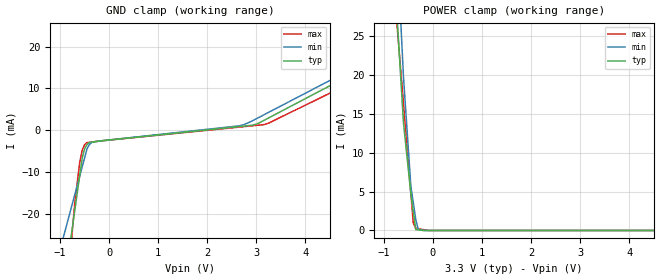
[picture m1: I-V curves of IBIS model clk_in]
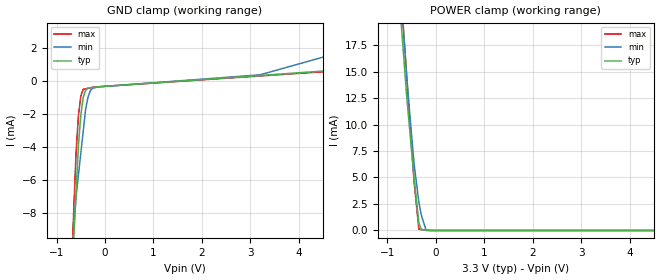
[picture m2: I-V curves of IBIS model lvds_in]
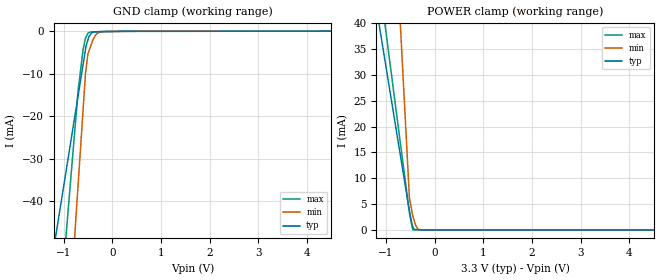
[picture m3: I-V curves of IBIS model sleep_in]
| Teraspeed (R) Labs.
| http://www.teraspeed.com
[IBIS Ver]   3.2
[Comment Char] |_char
[File Name]   dac5675aiphp.ibs
[File Rev]   3.0
[Date]   07-19-2011
[Notes]   Quality Check of this IBIS model: Model Passes IBIS Check
   Model parses into ICX IS. Simulation done with Hyperlynx.
   1. MIN TYP MAX information is based on Temprature and Voltage
   characteristics only.
   2. Package information extracted using Tektronix IConnect Software.
[Disclaimer]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
[Source]
| This model file was created by Teraspeed Consulting Group LLC
| (http://www.teraspeed.com/).
[Disclaimer]
| This product is designed as an aid for customers of Texas Instruments.
| No warranties, either expressed or implied, with respect to this third
| party software (if any) or with respect to its fitness for any
| particular purpose is claimed by Texas Instruments or the author. The
| software (if any) is provided solely on an "as is" basis. The entire
| risk as to its quality and performance is with the customer
[Copyright]
| (C) Copyright 2011 Texas Instruments Incorporated. All rights reserved.
| All other rights are reserved.
[Component]   DAC5675AIPHP
[Manufacturer] TI
[Package]
| 48-HTQFP
| variable   typ   min   max
R_pkg  1.000E-02  1.000E-02  1.000E-02
L_pkg  1.807E-09  1.620E-09  2.200E-09
C_pkg  6.730E-13  6.560E-13  7.110E-13
[Pin] signal_name  model_name  R_pin  L_pin C_pin
1   D13A   lvds_in   1.000E-02 2.200E-09 6.320E-13
2   D13B   lvds_in   1.000E-02 1.870E-09 7.110E-13
3   D12A   lvds_in   1.000E-02 1.790E-09 6.940E-13
4   D12B   lvds_in   1.000E-02 1.700E-09 6.770E-13
5   D11A   lvds_in   1.000E-02 1.660E-09 6.680E-13
6   D11B   lvds_in   1.000E-02 1.620E-09 6.560E-13
7   D10A   lvds_in   1.000E-02 1.620E-09 6.560E-13
8   D10B   lvds_in   1.000E-02 1.660E-09 6.680E-13
9   D9A   lvds_in   1.000E-02 1.700E-09 6.770E-13
10   D9B   lvds_in   1.000E-02 1.790E-09 6.940E-13
11   D8A   lvds_in   1.000E-02 1.870E-09 7.110E-13
12   D8B   lvds_in   1.000E-02 2.200E-09 6.320E-13
13   D7A   lvds_in   1.000E-02 2.200E-09 6.320E-13
14   D7B   lvds_in   1.000E-02 1.870E-09 7.110E-13
15   DVDD   POWER   1.000E-02 1.790E-09 6.940E-13
16   DGND   GND   1.000E-02 1.700E-09 6.770E-13
17   DVDD   POWER   1.000E-02 1.660E-09 6.680E-13
18   DGND   GND   1.000E-02 1.620E-09 6.560E-13
19   AGND   GND   1.000E-02 1.620E-09 6.560E-13
20   AVDD   POWER   1.000E-02 1.660E-09 6.680E-13
21   CLKC   clk_in   1.000E-02 1.700E-09 6.770E-13
22   CLK   clk_in   1.000E-02 1.790E-09 6.940E-13
23   D6A   lvds_in   1.000E-02 1.870E-09 7.110E-13
24   D6B   lvds_in   1.000E-02 2.200E-09 6.320E-13
25   D5A   lvds_in   1.000E-02 2.200E-09 6.320E-13
26   D5B   lvds_in   1.000E-02 1.870E-09 7.110E-13
27   D4A   lvds_in   1.000E-02 1.790E-09 6.940E-13
28   D4B   lvds_in   1.000E-02 1.700E-09 6.770E-13
29   D3A   lvds_in   1.000E-02 1.660E-09 6.680E-13
30   D3B   lvds_in   1.000E-02 1.620E-09 6.560E-13
31   D2A   lvds_in   1.000E-02 1.620E-09 6.560E-13
32   D2B   lvds_in   1.000E-02 1.660E-09 6.680E-13
33   D1A   lvds_in   1.000E-02 1.700E-09 6.770E-13
34   D1B   lvds_in   1.000E-02 1.790E-09 6.940E-13
35   D0A   lvds_in   1.000E-02 1.870E-09 7.110E-13
36   D0B   lvds_in   1.000E-02 2.200E-09 6.320E-13
37   SLEEP  sleep_in  1.000E-02 2.200E-09 6.320E-13
38   NC   NC   1.000E-02 1.870E-09 7.110E-13
39   BIASJ  term   1.000E-02 1.790E-09 6.940E-13
40   EXTIO  term   1.000E-02 1.700E-09 6.770E-13
41   AGND   GND   1.000E-02 1.660E-09 6.680E-13
42   AVDD   POWER   1.000E-02 1.620E-09 6.560E-13
43   IOUT1  analog   1.000E-02 1.620E-09 6.560E-13
44   IOUT2  analog   1.000E-02 1.660E-09 6.680E-13
45   AVDD   POWER   1.000E-02 1.700E-09 6.770E-13
46   AGND   GND   1.000E-02 1.790E-09 6.940E-13
47   AGND   GND   1.000E-02 1.870E-09 7.110E-13
48   AVDD   POWER   1.000E-02 2.200E-09 6.320E-13
[diff pin] inv_pin vdiff tdelay_typ tdelay_min tdelay_max
1   2  100mV  NA  NA  NA
3   4  100mV  NA  NA  NA
5   6  100mV  NA  NA  NA
7   8  100mV  NA  NA  NA
9   10  100mV  NA  NA  NA
11  12  100mV  NA  NA  NA
13  14  100mV  NA  NA  NA
21  22  400mV  NA  NA  NA
23  24  100mV  NA  NA  NA
25  26  100mV  NA  NA  NA
27  28  100mV  NA  NA  NA
29  30  100mV  NA  NA  NA
31  32  100mV  NA  NA  NA
33  34  100mV  NA  NA  NA
35  36  100mV  NA  NA  NA
[Series Pin Mapping]  pin_2  model_name
1   2  110ohm
3   4  110ohm
5   6  110ohm
7   8  110ohm
9   10  110ohm
11  12  110ohm
13   14 110ohm
23  24  110ohm
25 26 110ohm
27  28  110ohm
29  30  110ohm
31  32  110ohm
33  34  110ohm
35  36  110ohm
[Model] 110ohm
Model_type Series
| variable   typ   min   max
C_comp   0.00000pF 0.00000pF 0.00000pF
[Voltage Range] 3.30000V 3.15000V 3.45000V
[R Series] 110  90  132
[Model] analog
Model_type Terminator
C_comp  0.00000pF 0.00000pF 0.00000pF
| variable   typ   min   max
[Voltage Range]   3.3000V  3.1500V  3.4500V
[POWER Clamp Reference]  3.3000V  3.1500V  3.4500V
[GND Clamp Reference]   0.0000V  0.0000V  0.0000V
[Temperature Range]   25   125   -55
[Model] term
Model_type Terminator
C_comp  0.00000pF 0.00000pF 0.00000pF
| variable   typ   min   max
[Voltage Range]   3.3000V  3.1500V  3.4500V
[POWER Clamp Reference]  3.3000V  3.1500V  3.4500V
[GND Clamp Reference]   0.0000V  0.0000V  0.0000V
[Temperature Range]   25   125   -55
| Models and submodels in the file (6): 110ohm (Series), analog (Terminator), clk_in (Input), lvds_in (Input), sleep_in (Input), term (Terminator)
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[Model] clk_in
Model_type Input
Vinl = 1.60000V
Vinh = 2.40000V
C_comp 2.00000pF 2.00000pF 2.00000pF
| variable typ   min   max
[Voltage Range] 3.30000V 3.15000V 3.45000V
[POWER Clamp Reference] 3.30000V 3.15000V 3.45000V
[GND Clamp Reference] 0.00000V 0.00000V 0.00000V
[Temperature Range]   25   125   -55
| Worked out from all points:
|   POWER clamp passes 1 mA (typ) near -0.37 V on its own axis
[GND Clamp]
-3.3V     -235.6mA   -129.6mA   -365.3mA
-700mV    -19.2mA    -15.43mA   -17.4mA
-600mV    -10.88mA   -11.04mA   -7.717mA
-550mV    -6.717mA   -8.845mA   -4.83mA
-500mV    -4.508mA   -6.651mA   -3.457mA
-450mV    -3.391mA   -4.456mA   -3.007mA
-350mV    -2.892mA   -2.948mA   -2.854mA
-175mV    -2.606mA   -2.578mA   -2.605mA
2.65V     831.8uA    1.01mA     703.4uA
3V        1.422mA    2.714mA    1.113mA
3.25V     2.907mA    4.243mA    1.664mA
6.6V      23.58mA    24.73mA    20.89mA
[POWER Clamp]
-3.3V     296.9mA    367.3mA    224.2mA
-600mV    13.87mA    19.81mA    16.36mA
-450mV    4.767mA    5.737mA    4.815mA
-400mV    2.442mA    3.586mA    966uA
-350mV    117.3uA    1.434mA    290uA
-300mV    83.81uA    144.2uA    232uA
-200mV    16.76uA    0A         116uA
-75mV     0A         0A         0A
6.6V      0A         0A         0A
[Model] lvds_in
Model_type Input
Vinl = 1100.00mV
Vinh = 1.3000V
C_comp 2.00000pF 2.00000pF 2.00000pF
| variable typ   min   max
[Voltage Range] 3.30000V 3.15000V 3.45000V
[POWER Clamp Reference] 3.30000V 3.15000V 3.45000V
[GND Clamp Reference] 0.00000V 0.00000V 0.00000V
[Temperature Range]   25   125   -55
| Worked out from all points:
|   GND clamp passes 1 mA (typ) near -0.45 V on its own axis
|   POWER clamp passes 1 mA (typ) near -0.36 V on its own axis
[GND Clamp]
-3.3V     -164.4mA   -124.7mA   -204.6mA
-600mV    -6.813mA   -7.033mA   -4.418mA
-550mV    -3.894mA   -5.7mA     -2.115mA
-500mV    -2.059mA   -4.367mA   -909.1uA
-450mV    -993.7uA   -3.034mA   -502.3uA
-400mV    -558.2uA   -1.701mA   -472.1uA
-350mV    -428.5uA   -951.4uA   -441.8uA
-300mV    -409.1uA   -580.5uA   -411.6uA
-250mV    -389.8uA   -435.3uA   -381.4uA
-125mV    -350.5uA   -353.8uA   -346.8uA
3.2V      329.9uA    370.1uA    300.6uA
6.6V      1.026mA    3.158mA    962.6uA
[POWER Clamp]
-3.3V     176.5mA    194.6mA    191.7mA
-600mV    12.58mA    14.34mA    14.51mA
-450mV    5.01mA     6.33mA     4.67mA
-350mV    695uA      2.654mA    108.7uA
-300mV    102.3uA    1.461mA    86.96uA
-200mV    34.09uA    0A         43.48uA
6.6V      0A         0A         0A
[Model] sleep_in
Model_type Input
Vinl = 800.000mV
Vinh = 2.00000V
C_comp 2.00000pF 2.00000pF 2.00000pF
| variable typ   min   max
[Voltage Range] 3.30000V 3.15000V 3.45000V
[POWER Clamp Reference] 3.30000V 3.15000V 3.45000V
[GND Clamp Reference] 0.00000V 0.00000V 0.00000V
[Temperature Range]   25   125   -55
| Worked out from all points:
|   GND clamp passes 1 mA (typ) near -0.47 V on its own axis
|   POWER clamp passes 1 mA (typ) near -0.46 V on its own axis
[GND Clamp]
-3.3V     -201.7mA   -485.5mA   -371.5mA
-700mV    -15.05mA   -35.93mA   -13.79mA
-600mV    -7.869mA   -18.63mA   -4.318mA
-550mV    -4.279mA   -9.988mA   -1.613mA
-540mV    -3.561mA   -9.043mA   -1.378mA
-500mV    -2.006mA   -5.265mA   -435.6uA
-480mV    -1.228mA   -4.628mA   -308.6uA
-450mV    -766.9uA   -3.673mA   -118.2uA
-400mV    -214.7uA   -2.081mA   -100.5uA
-300mV    -86.34uA   -392.9uA   -65.18uA
-125mV    -25.47uA   -20.9uA    -23.48uA
6.6V      82.28uA    83.68uA    70.72uA
[POWER Clamp]
-3.3V     165mA      507.1mA    205mA
-650mV    11.19mA    29.61mA    12.75mA
-520mV    3.643mA    6.191mA    3.316mA
-460mV    797.3uA    3.102mA    420.8uA
-450mV    618.1uA    2.662mA    59.81uA
-420mV    80.18uA    1.724mA    53.83uA
-400mV    72.55uA    1.099mA    49.84uA
-350mV    53.45uA    182.4uA    39.87uA
-250mV    15.27uA    12.34uA    19.94uA
6.6V      0A         0A         0A
